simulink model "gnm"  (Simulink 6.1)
settings: Solver=ode45  StartTime=0.0  StopTime=Tstop  MaxStep=step_max  RelTol=1e-3
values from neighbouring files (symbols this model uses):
  CE = 2*pi*CM    (= 240.017678734)    [gnm_i.m]
  CM = 38.2    [gnm_i.m]
  J = 0.012    [gnm_i.m]
  MW = 10    [gnmbeobreg_i.m]    (also in gnmbeob_i.m; gnmregn_i.m = 100; gnm_i.m = 0; lsg_gnmregnss_ini.m = 100)
  PsiN = 0.04    [gnm_i.m]
  RA = 0.250    (= 0.25)    [gnm_i.m]
  T_MW = 0.4    [gnmbeobreg_i.m]    (also in gnmbeob_i.m; gnmregn_i.m = 0.1; gnm_i.m = 0; lsg_gnmregnss_ini.m = 0.1)
  TA = LA / RA    (= 0.016)    [gnm_i.m]
  Tsprung = 0    [gnm_i.m]
  UAsoll = 50    [gnm_i.m]

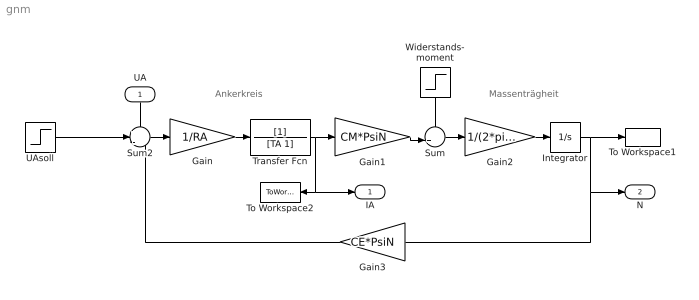
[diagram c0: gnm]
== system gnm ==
  note: Massenträgheit
  note: Ankerkreis
  UA : Inport  Orientation=down  Port=1  LatchInput=off
  Gain : Gain  Gain=1/RA
  Gain1 : Gain  Gain=CM*PsiN
  Gain2 : Gain  Gain=1/(2*pi*J)
  Gain3 : Gain  Orientation=left  Gain=CE*PsiN
  Integrator : Integrator
  Sum : Sum  Inputs=-+|
  Sum2 : Sum  Inputs=++-
  To Workspace1 : ToWorkspace  VariableName=N  SampleTime=-1  SaveFormat=Array
  To Workspace2 : ToWorkspace  VariableName=IA  SampleTime=-1  SaveFormat=Array
  Transfer Fcn : TransferFcn  Denominator=[TA 1]
  UAsoll : Step  Time=Tsprung  After=UAsoll  SampleTime=0
  Widerstands- moment : Step  Orientation=down  Time=T_MW  After=MW  SampleTime=0
  IA : Outport
  N : Outport  Port=2
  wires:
  Gain/1 -> Transfer Fcn/1
  Sum2/1 -> Gain/1
  Gain1/1 -> Sum/2
  Widerstands- moment/1 -> Sum/1
  Sum/1 -> Gain2/1
  Gain2/1 -> Integrator/1
  Integrator/1 -> To Workspace1/1, N/1, Gain3/1
  UA/1 -> Sum2/1
  Gain3/1 -> Sum2/3
  Transfer Fcn/1 -> Gain1/1, To Workspace2/1, IA/1
  UAsoll/1 -> Sum2/2
